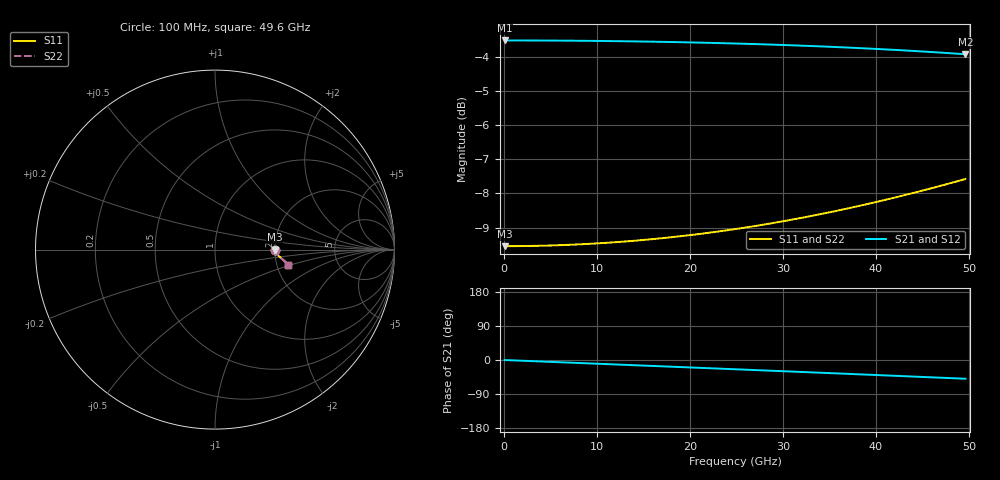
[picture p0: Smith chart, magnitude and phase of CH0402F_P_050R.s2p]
# GHz S RI R 50
! S-Parameters data
! Freq  reS11  imS11  reS21  imS21  reS12  imS12  reS22  imS22
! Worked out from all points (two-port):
!   100 points, 100 MHz to 49.6 GHz, reference 50 ohm
!   highest |S21| = -3.52 dB at 100 MHz (marker M1); lowest = -3.9 dB at 49.6 GHz (marker M2)
!   |S21| within 3 dB of the highest: start of sweep to end of sweep
!   lowest |S11| = -9.5 dB at 100 MHz (marker M3), VSWR 2.00, Z = 100 - j0.0267 ohm
!   |S11| at or under -10 dB: nowhere
!   |S22| runs from -9.5 to -7.6 dB; largest |S21 - S12| = 0
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0.1  0.3333 -0.000119  0.6667 -0.00114  0.6667 -0.00114  0.3333 -0.000119
2.1  0.3335 -0.00249  0.6662 -0.0239  0.6662 -0.0239  0.3335 -0.00249
4.1  0.3338 -0.00488  0.6649 -0.0466  0.6649 -0.0466  0.3338 -0.00488
6.1  0.3344 -0.00727  0.6627 -0.0693  0.6627 -0.0693  0.3344 -0.00727
8.6  0.3355 -0.0103  0.6587 -0.0975  0.6587 -0.0975  0.3355 -0.0103
10.6  0.3366 -0.0128  0.6546 -0.1199  0.6546 -0.1199  0.3366 -0.0128
12.6  0.3379 -0.0152  0.6496 -0.1421  0.6496 -0.1421  0.3379 -0.0152
14.6  0.3395 -0.0178  0.6438 -0.1642  0.6438 -0.1642  0.3395 -0.0178
16.6  0.3414 -0.0204  0.6371 -0.186  0.6371 -0.186  0.3414 -0.0204
18.6  0.3435 -0.0231  0.6296 -0.2075  0.6296 -0.2075  0.3435 -0.0231
20.6  0.3458 -0.0258  0.6213 -0.2288  0.6213 -0.2288  0.3458 -0.0258
22.6  0.3484 -0.0286  0.6121 -0.2498  0.6121 -0.2498  0.3484 -0.0286
25.1  0.352 -0.0323  0.5995 -0.2754  0.5995 -0.2754  0.352 -0.0323
27.1  0.3552 -0.0354  0.5885 -0.2955  0.5885 -0.2955  0.3552 -0.0354
29.1  0.3586 -0.0386  0.5767 -0.3152  0.5767 -0.3152  0.3586 -0.0386
33.1  0.3663 -0.0456  0.5507 -0.3531  0.5507 -0.3531  0.3663 -0.0456
37.1  0.3751 -0.0533  0.5218 -0.3889  0.5218 -0.3889  0.3751 -0.0533
39.1  0.3799 -0.0575  0.5062 -0.4058  0.5062 -0.4058  0.3799 -0.0575
41.6  0.3863 -0.0632  0.4858 -0.4262  0.4858 -0.4262  0.3863 -0.0632
45.6  0.3973 -0.0731  0.4509 -0.4564  0.4509 -0.4564  0.3973 -0.0731
47.6  0.4032 -0.0786  0.4326 -0.4704  0.4326 -0.4704  0.4032 -0.0786
49.6  0.4093 -0.0845  0.4136 -0.4836  0.4136 -0.4836  0.4093 -0.0845
